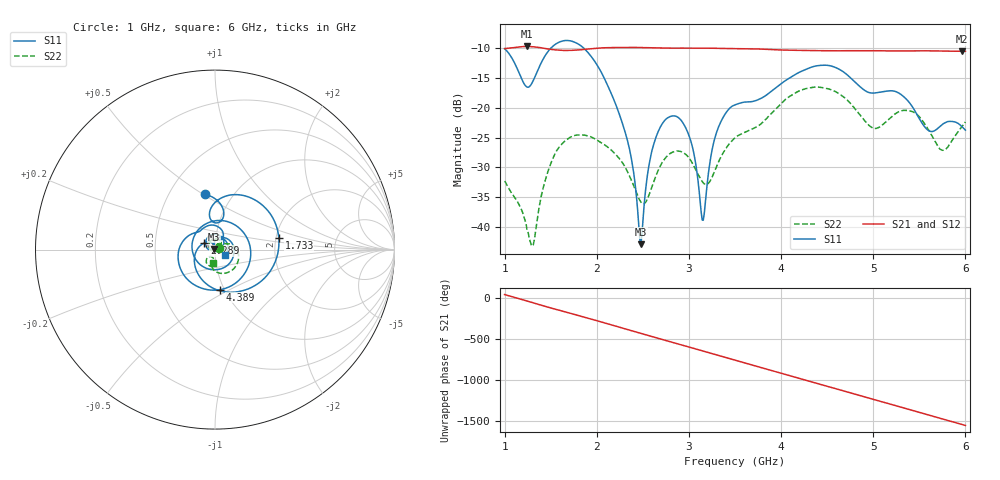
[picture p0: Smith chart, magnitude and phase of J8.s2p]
!Agilent Technologies,E8364B,MY43040528,A.07.50.67
!Agilent E8364B: A.07.50.67
!Date: Sunday, March 01, 2026 19:08:56
!Correction: S11(Full 2 Port(1,2))
!S21(Full 2 Port(1,2))
!S12(Full 2 Port(1,2))
!S22(Full 2 Port(1,2))
!S2P File: Measurements: S11, S21, S12, S22:
# Hz S  dB  R 50
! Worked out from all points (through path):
!   451 points, 1 GHz to 6 GHz, reference 50 ohm
!   highest |S21| = -9.71 dB at 1.244 GHz (marker M1); lowest = -10.5 dB at 5.967 GHz (marker M2)
!   group delay of S21, straight-line fit = 889 ps
!   lowest |S11| = -42.9 dB at 2.478 GHz (marker M3), VSWR 1.01, Z = 49.4 + j0.402 ohm
!   |S11| at or under -10 dB: start of sweep to 1.501 GHz; 1.86 GHz to end of sweep
!   |S22| runs from -43.2 to -16.5 dB; largest |S21 - S12| = 0.0014
!   S11 on the Smith chart (normalised r, x): 1 GHz: 0.74, +0.51; 1.733 GHz: 2.08, +0.30; 2.289 GHz: 0.89, +0.07; 4.389 GHz: 0.95, -0.45; 6 GHz: 1.12, -0.06
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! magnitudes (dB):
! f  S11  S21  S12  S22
! 1 GHz  -10.1  -10.1  -10.1  -32.3
! 1.244 GHz  -16.5  -9.7  -9.7  -40.7
! 1.311 GHz  -15.4  -9.8  -9.8  -43.0
! 1.489 GHz  -10.2  -10.2  -10.2  -29.9
! 1.733 GHz  -8.8  -10.4  -10.4  -24.8
! 1.844 GHz  -9.8  -10.2  -10.3  -24.6
! 2.289 GHz  -23.1  -9.9  -9.9  -29.5
! 2.389 GHz  -29.7  -9.9  -9.9  -32.6
! 2.478 GHz  -42.9  -9.9  -9.9  -35.8
! 2.567 GHz  -29.6  -9.9  -9.9  -34.6
! 2.667 GHz  -24.0  -10.0  -10.0  -30.5
! 2.956 GHz  -23.1  -10.0  -10.0  -27.7
! 3.156 GHz  -38.9  -10.0  -10.0  -32.6
! 3.289 GHz  -24.7  -10.0  -10.0  -30.3
! 3.5 GHz  -19.5  -10.1  -10.1  -25.0
! 4.344 GHz  -13.1  -10.4  -10.4  -16.6
! 4.389 GHz  -13.0  -10.4  -10.4  -16.5
! 5.167 GHz  -17.2  -10.5  -10.5  -22.0
! 5.444 GHz  -20.3  -10.4  -10.5  -20.8
! 5.756 GHz  -22.7  -10.5  -10.5  -27.1
! 5.967 GHz  -23.2  -10.5  -10.5  -23.1
! 6 GHz  -23.7  -10.5  -10.5  -22.4
